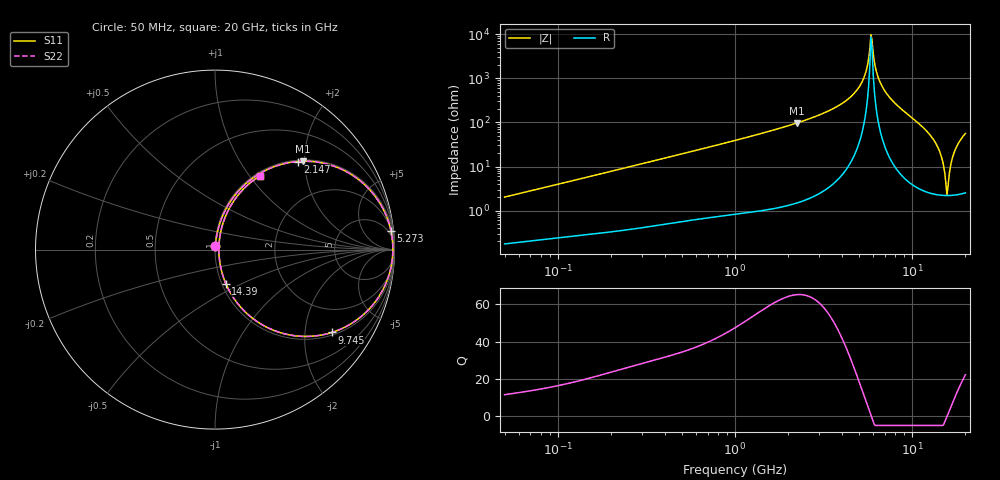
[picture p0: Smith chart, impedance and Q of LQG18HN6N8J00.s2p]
!Murata Part Number: LQG18HN6N8J00
!These Parameters are Measured in Series Mode Connection
!  o--[Z]--o
!Port1  Port2
!  o-------o
!Freq. Start=50[MHz] Stop=20[GHz], 401[Steps]
# Hz S RI R 50
!Freq.(Hz) S11(Real) S11(Imag) S21(Real) S21(Imag) S12(Real) S12(Imag) S22(Real) S22(Imag)
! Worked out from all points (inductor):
!   401 points, 50 MHz to 20 GHz, reference 50 ohm
!   read as one part in series: L = 6.38 nH near 51.52 MHz
!   highest Q = 65.2 at 2.245 GHz (marker M1), where L = 6.92 nH
!   self-resonance near 5.856 GHz
!   S11 on the Smith chart (normalised r, x): 50 MHz: 1.00, +0.04; 2.147 GHz: 1.03, +1.84; 5.273 GHz: 2, +18; 9.745 GHz: 1.08, -2.75; 14.39 GHz: 1.04, -0.41; 20 GHz: 1.05, +1.12
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5e7  0.00216 0.0201  0.9978 -0.0201  0.9978 -0.0201  0.00216 0.0201
1.364002e8  0.0056 0.0531  0.9944 -0.0531  0.9944 -0.0531  0.0056 0.0531
3.721004e8  0.0247 0.1398  0.9753 -0.1398  0.9753 -0.1398  0.0247 0.1398
1e9  0.1372 0.3337  0.8628 -0.3337  0.8628 -0.3337  0.1372 0.3337
2.146657e9  0.4598 0.4907  0.5402 -0.4907  0.5402 -0.4907  0.4598 0.4907
2.245319e9  0.4882 0.4922  0.5118 -0.4922  0.5118 -0.4922  0.4882 0.4922
2.728004e9  0.6189 0.4778  0.3811 -0.4778  0.3811 -0.4778  0.6189 0.4778
4.212059e9  0.8973 0.2906  0.1027 -0.2906  0.1027 -0.2906  0.8973 0.2906
5.273168e9  0.98 0.1064  0.02 -0.1064  0.02 -0.1064  0.98 0.1064
5.515528e9  0.9873 0.0638  0.0127 -0.0638  0.0127 -0.0638  0.9873 0.0638
5.769027e9  0.9908 0.0197  0.00917 -0.0197  0.00917 -0.0197  0.9908 0.0197
5.944466e9  0.991 -0.0104  0.00904 0.0104  0.00904 0.0104  0.991 -0.0104
6.503449e9  0.9796 -0.1031  0.0204 0.1031  0.0204 0.1031  0.9796 -0.1031
7.442007e9  0.9246 -0.2433  0.0754 0.2433  0.0754 0.2433  0.9246 -0.2433
9.745021e9  0.6504 -0.4618  0.3496 0.4618  0.3496 0.4618  0.6504 -0.4618
1.238412e10  0.2555 -0.4144  0.7445 0.4144  0.7445 0.4144  0.2555 -0.4144
1.438523e10  0.0603 -0.1898  0.9397 0.1898  0.9397 0.1898  0.0603 -0.1898
1.573793e10  0.0215 -0.0036  0.9785 0.0036  0.9785 0.0036  0.0215 -0.0036
1.621653e10  0.0253 0.0604  0.9747 -0.0604  0.9747 -0.0604  0.0253 0.0604
1.670968e10  0.0374 0.1231  0.9626 -0.1231  0.9626 -0.1231  0.0374 0.1231
1.747767e10  0.0704 0.212  0.9296 -0.212  0.9296 -0.212  0.0704 0.212
2e10  0.2501 0.4111  0.7499 -0.4111  0.7499 -0.4111  0.2501 0.4111
